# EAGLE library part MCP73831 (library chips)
Description: Device for MCP73831, a battery charge controller from Microchip.
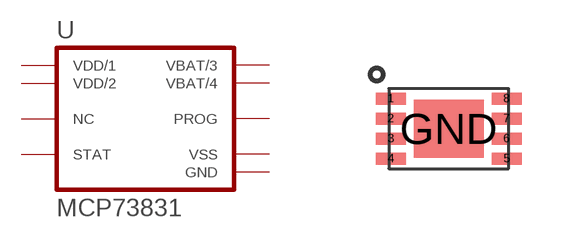
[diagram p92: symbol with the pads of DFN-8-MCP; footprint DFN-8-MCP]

Designator prefix U

## MCP73831 (DATASHEET: http://ww1.microchip.com/downloads/en/DeviceDoc/20001984g.pdf; DESCRIPTION: IC CONTROLLER LI-ION 4.2V 8DFN; DIGIKEY: MCP73831T-2ACI/MCCT-ND; MANUFACTURER: Microchip Technology; MOUSER: 579-MCP73832T-2ACIMC; MPN: MCP73831T-2ACI/MC)  [DFN-8-MCP]
1  VDD/1  pwr
2  VDD/2  pwr
3  VBAT/3  pwr
4  VBAT/4  pwr
5  STAT
6  VSS  pwr
7  NC  nc
8  PROG
GND  GND  pwr

## Footprint DFN-8-MCP (pad centres in mm)
Description: Package for the MCP73831, a battery charge controller from Microchip.
smd 0.75 x 0.3: 1 -1.45,0.75; 2 -1.45,0.25; 3 -1.45,-0.25; 4 -1.45,-0.75; 5 1.45,-0.75; 6 1.45,-0.25; 7 1.45,0.25; 8 1.45,0.75
smd 1.75 x 1.45: GND 0,0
